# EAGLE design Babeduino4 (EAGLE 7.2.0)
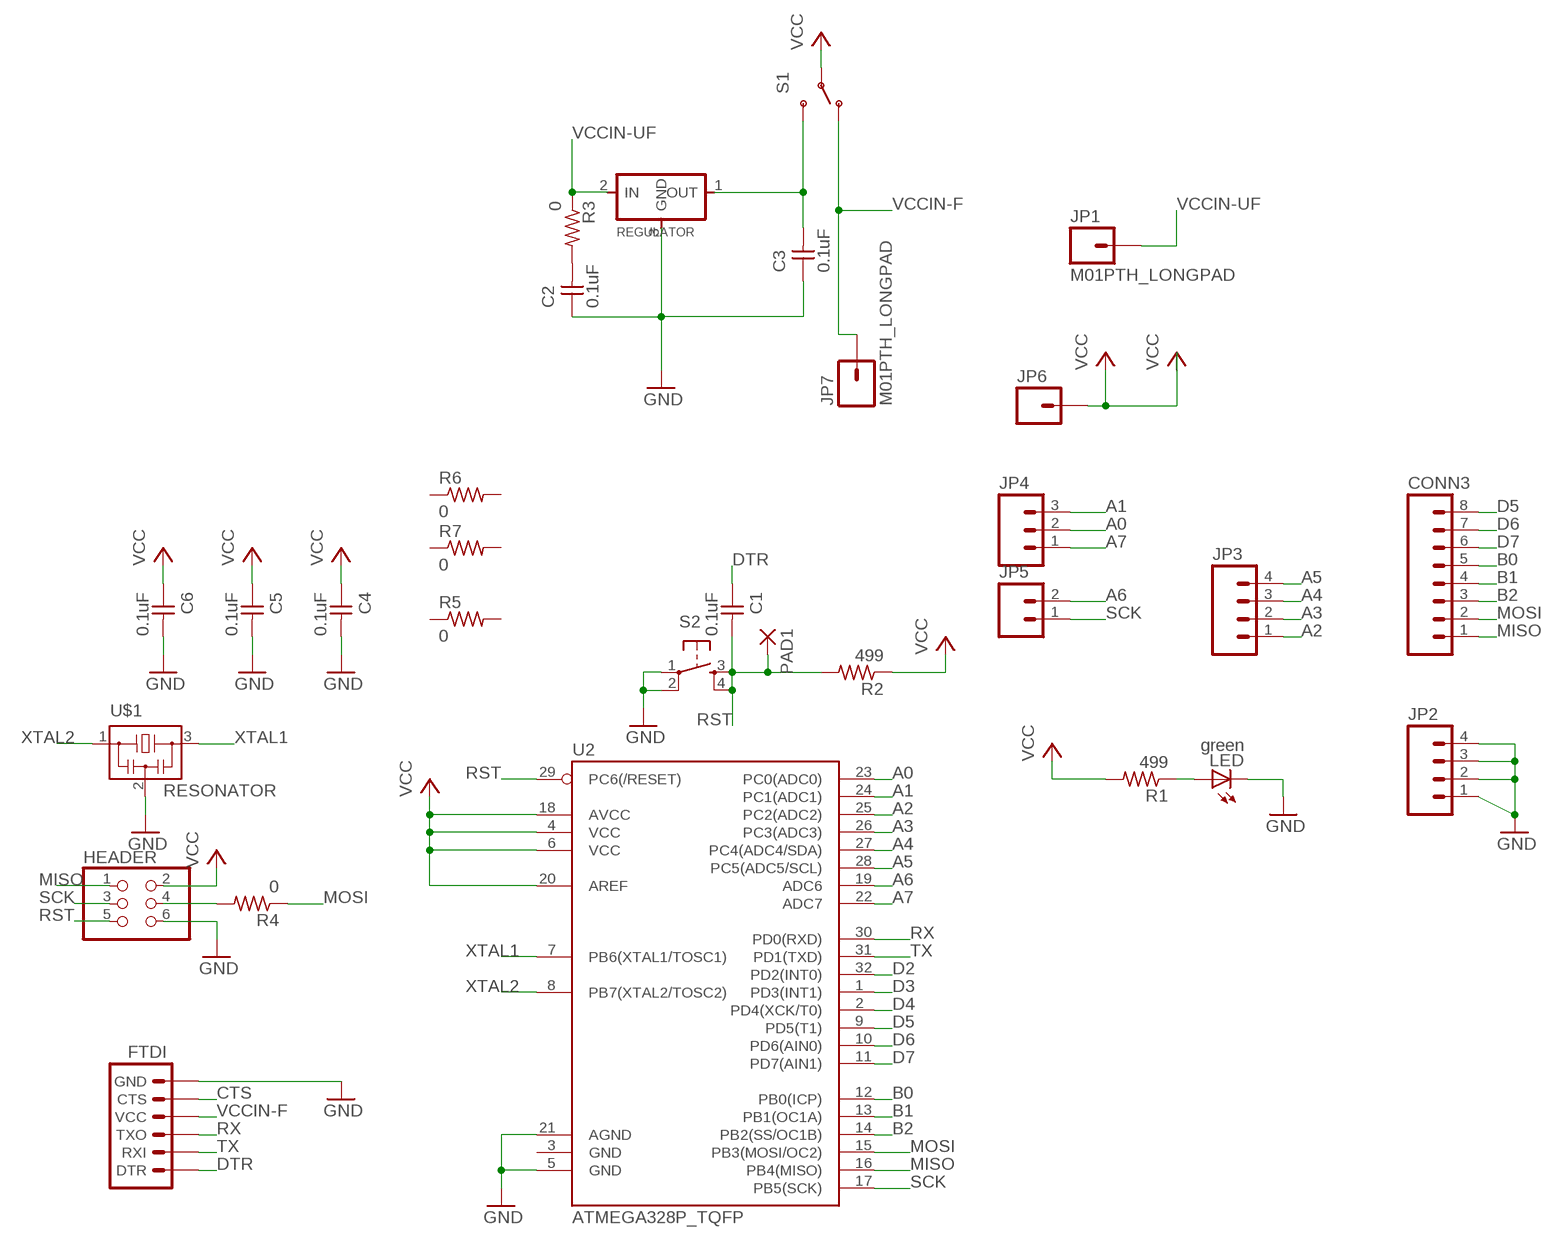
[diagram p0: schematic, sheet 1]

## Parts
C1  0.1uF  UNPOLARIZED_CAPACITOR1206  [1206]
C2  0.1uF  UNPOLARIZED_CAPACITOR1206  [1206]
C3  0.1uF  UNPOLARIZED_CAPACITOR1206  [1206]
C4  0.1uF  UNPOLARIZED_CAPACITOR1206  [1206]
C5  0.1uF  UNPOLARIZED_CAPACITOR1206  [1206]
C6  0.1uF  UNPOLARIZED_CAPACITOR1206  [1206]
CONN3  M08LONGPADS  [1X08_LONGPADS]
FTDI  ARDUINO_SERIAL_PROGRAMSMD  [1X06-SMD]
HEADER  PINHD-2X3-SMD  [2X03SMD]
JP1  M01PTH_LONGPAD  [1X01_LONGPAD]
JP2  M04LONGPADS  [1X04_LONGPADS]
JP3  M04LONGPADS  [1X04_LONGPADS]
JP4  M03LONGPADS  [1X03_LONGPADS]
JP5  M02  [1X02_LONGPADS]
JP6  M01PTH_LONGPAD  [1X01_LONGPAD]
JP7  M01PTH_LONGPAD  [1X01_LONGPAD]
LED  green  LED1206  [1206]
PAD1  WIREPAD2,54/0,9  [2,54/0,9]
R1  499  RESISTOR1206  [1206]
R2  499  RESISTOR1206  [1206]
R3  0  RESISTOR1206  [1206]
R4  0  RESISTOR1206  [1206]
R5  0  RESISTOR1206  [1206]
R6  0  RESISTOR1206  [1206]
R7  0  RESISTOR1206  [1206]
REGULATOR  REGULATORSOT23  [SOT23]
S1  SWITCH-SPDTSMD2  [SWITCH-SPDT-SMD]
S2  6MM_SWITCH6MM_SWITCH  [6MM_SWITCH]
U2  ATMEGA328P_TQFP  [TQFP32-08]
U$1  RESONATOR  [EFOBM]

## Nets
A0: JP4.2 U2.23(PC0(ADC0))
A1: JP4.3 U2.24(PC1(ADC1))
A2: JP3.1 U2.25(PC2(ADC2))
A3: JP3.2 U2.26(PC3(ADC3))
A4: JP3.3 U2.27(PC4(ADC4/SDA))
A5: JP3.4 U2.28(PC5(ADC5/SCL))
A6: JP5.2 U2.19(ADC6)
A7: JP4.1 U2.22(ADC7)
B0: CONN3.5 U2.12(PB0(ICP))
B1: CONN3.4 U2.13(PB1(OC1A))
B2: CONN3.3 U2.14(PB2(SS/OC1B))
CTS: FTDI.5(CTS)
D2: U2.32(PD2(INT0))
D3: U2.1(PD3(INT1))
D4: U2.2(PD4(XCK/T0))
D5: CONN3.8 U2.9(PD5(T1))
D6: CONN3.7 U2.10(PD6(AIN0))
D7: CONN3.6 U2.11(PD7(AIN1))
DTR: C1.1 FTDI.1(DTR)
GND: C2.1 C3.1 C4.2 C5.2 C6.2 FTDI.6(GND) HEADER.6 JP2.1 JP2.2 JP2.3 JP2.4 LED.2(C) REGULATOR.3(GND) S2.1(P) S2.2(P1) U2.5(GND) U2.21(AGND) U$1.2
MISO: CONN3.1 HEADER.1 U2.16(PB4(MISO))
MOSI: CONN3.2 R4.1 U2.15(PB3(MOSI/OC2))
N$1: LED.1(A) R1.1
N$2: HEADER.4 R4.2
N$3: C2.2 R3.2
N$4: C3.2 REGULATOR.1(OUT) S1.3(S)
RST: C1.2 HEADER.5 PAD1.1(P) R2.2 S2.3(S) S2.4(S1) U2.29(PC6(/RESET))
RX: FTDI.3(TXO) U2.30(PD0(RXD))
SCK: HEADER.3 JP5.1 U2.17(PB5(SCK))
TX: FTDI.2(RXI) U2.31(PD1(TXD))
VCC: C4.1 C5.1 C6.1 HEADER.2 JP6.1 R1.2 R2.1 S1.2(P) U2.4(VCC) U2.6(VCC) U2.18(AVCC) U2.20(AREF)
VCCIN-F: FTDI.4(VCC) JP7.1 S1.1(O)
VCCIN-UF: JP1.1 R3.1 REGULATOR.2(IN)
XTAL1: U2.7(PB6(XTAL1/TOSC1)) U$1.3
XTAL2: U2.8(PB7(XTAL2/TOSC2)) U$1.1
Unconnected: R5.1 R5.2 R6.1 R6.2 R7.1 R7.2 U2.3(GND)

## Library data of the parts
C1-C6 = 01_FAB_Hello:UNPOLARIZED_CAPACITOR: unpolarized_capacitor
CONN3 = 01_SparkFun:M08: Header 8 Standard 8-pin 0.1" header. Use with straight break away headers (SKU : PRT-00116), right angle break away headers (PRT-00553), swiss pins (PRT-00743), machine pins (PRT-00117), and female headers (PRT-00115).
FTDI = SparkFun-Connectors:ARDUINO_SERIAL_PROGRAM: FTDI connector footprints; PROD_ID: CONN-08971
HEADER = 01_FAB_Hello:PINHD-2X3-SMD: PIN HEADER
JP1 JP6 JP7 = 01_SparkFun:M01: Header 1
JP2 JP3 = 01_SparkFun:M04: Header 4 Standard 4-pin 0.1" header. Use with straight break away headers (SKU : PRT-00116), right angle break away headers (PRT-00553), swiss pins (PRT-00743), machine pins (PRT-00117), and female headers (PRT-00115). Molex polarized connector foot print use with SKU : PRT-08231 with associated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
JP4 = SparkFun-Connectors:M03: Header 3 Standard 3-pin 0.1" header. Use with straight break away headers (SKU : PRT-00116), right angle break away headers (PRT-00553), swiss pins (PRT-00743), machine pins (PRT-00117), and female headers (PRT-00115). Molex polarized connector foot print use with SKU : PRT-08232 with associated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
JP5 = 01_SparkFun:M02: Header 2
LED = 01_FAB_Hello:LED
PAD1 = wirepad:WIREPAD: Wire PAD connect wire on PCB
R1-R7 = 01_FAB_Hello:RESISTOR
REGULATOR = 01_fab:REGULATOR
S1 = SparkFun-Electromechanical:SWITCH-SPDT: SPDT Switch Simple slide switch, Spark Fun Electronics SKU : COM-00102 DPDT SMT slide switch, AYZ0202, SWCH-08179
S2 = 01_FAB_Hello:6MM_SWITCH: OMRON SWITCH
U2 = SparkFun-DigitalIC:ATMEGA328P_TQFP; PROD_ID: IC-09069
U$1 = 01_fab:RESONATOR

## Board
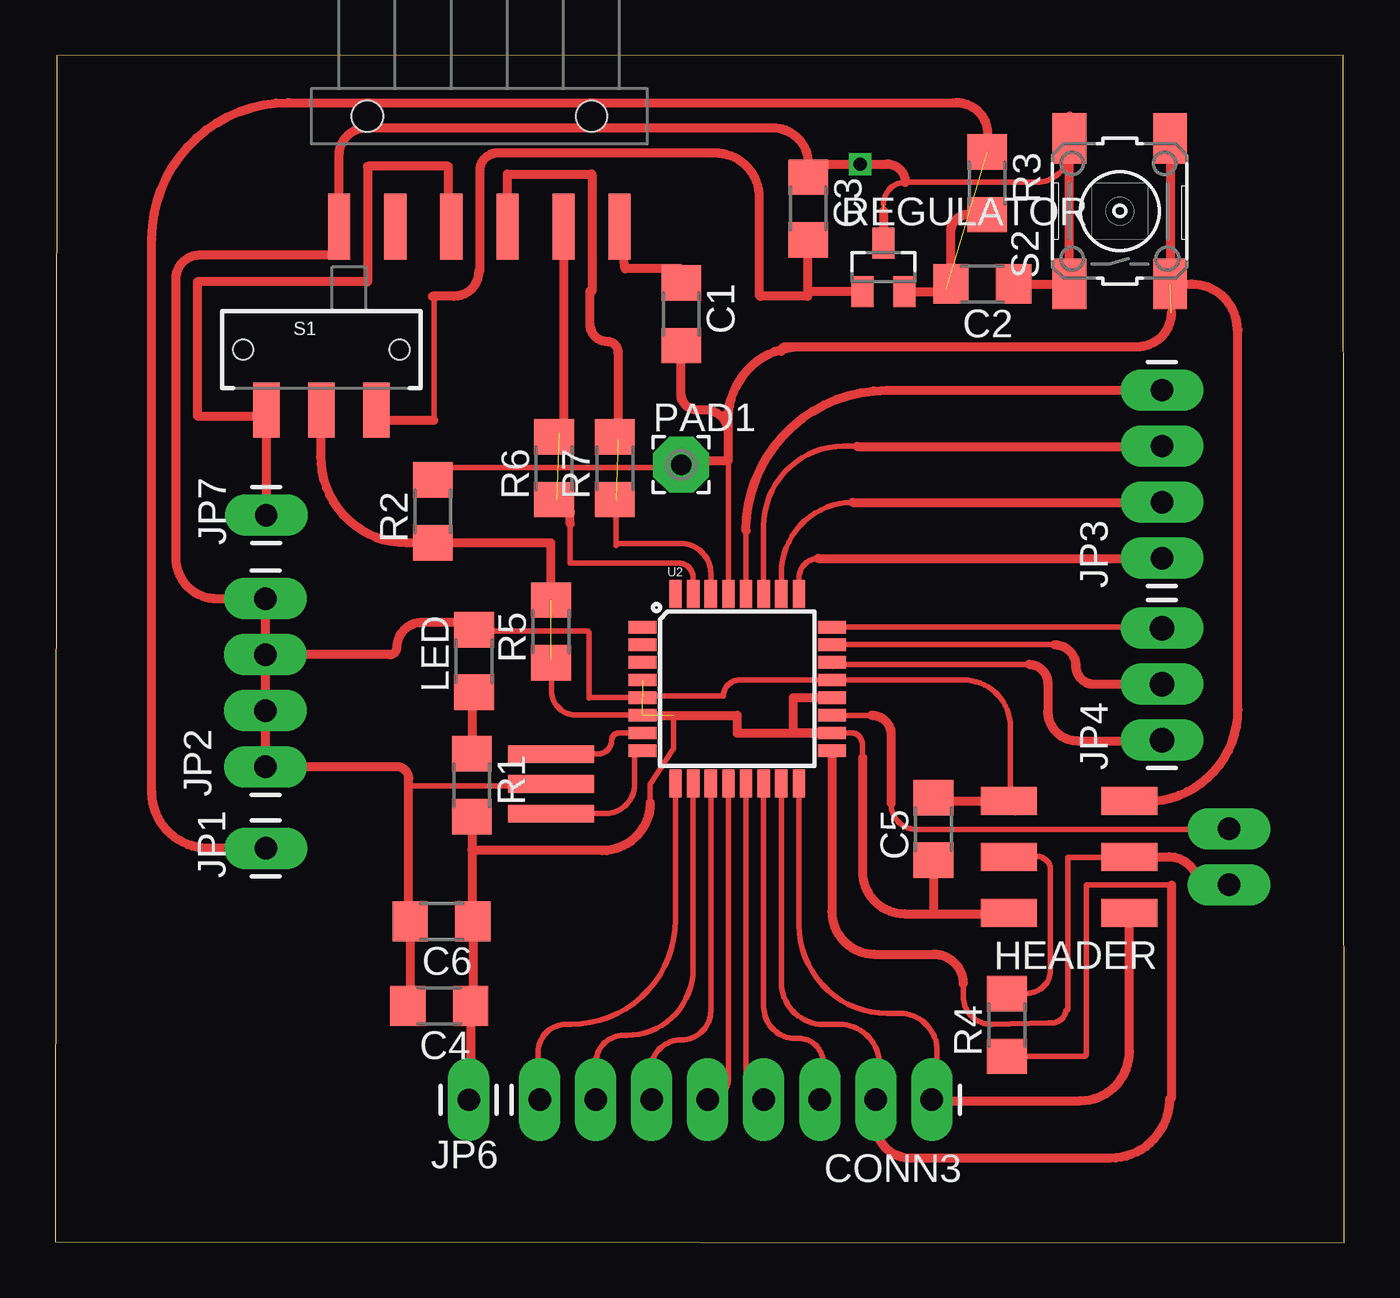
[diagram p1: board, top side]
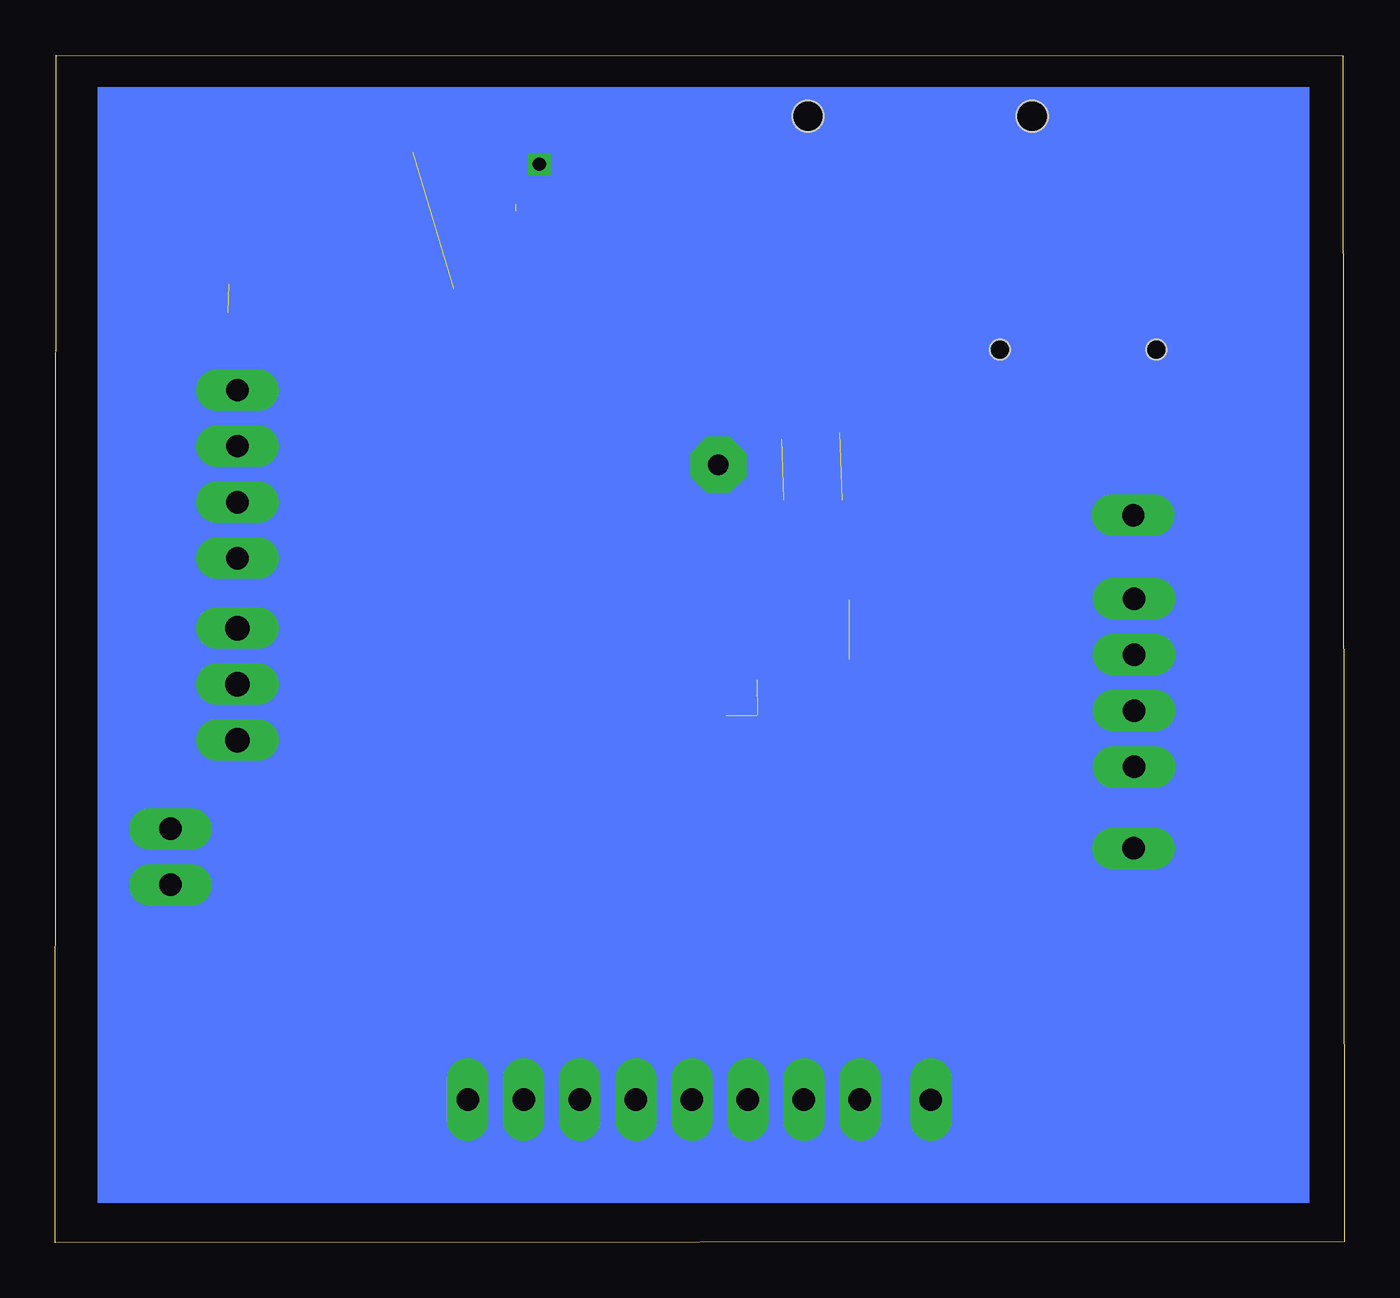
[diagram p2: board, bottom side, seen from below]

Size 58.45 x 53.84 mm. Coordinates in mm from the lower left corner, seen from the top.
Outline: 0,0.04 58.45,0 58.39,53.84 0.08,53.81 0,0.04
Copper layers (1*16): Top 0.035mm / dielectric 1.5mm / Bottom 0.035mm
Design rules "fabmodule": minimum track width 10mil, minimum drill 0.4mm, track to track 0.42mm, track to pad 0.42mm, pad to pad 0.42mm, via to via 0.42mm, smd to smd 0.42mm, copper to edge 40mil, drill to drill 0.8mm, minimum pad ring 10mil, minimum via ring 8mil, stop-mask expansion 4mil, vias tented up to drill 0mil, thermal gap 10mil

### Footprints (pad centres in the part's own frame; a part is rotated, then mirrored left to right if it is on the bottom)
1206 = smd 1.6 x 1.803: 1 -1.422,0; 2 1.422,0
1X08_LONGPADS = drill 1.016 pad 1.88 long: 1 0,0; 2 2.54,0; 3 5.08,0; 4 7.62,0; 5 10.16,0; 6 12.7,0; 7 15.24,0; 8 17.78,0
1X06-SMD = smd 1 x 3: 1 -6.35,5; 2 -3.81,5; 3 -1.27,5; 4 1.27,5; 5 3.81,5; 6 6.35,5 | hole 1.4: -5.08,0; 5.08,0
2X03SMD = smd 2.54 x 1.27: 1 -2.54,2.54; 2 2.92,2.54; 3 -2.54,0; 4 2.92,0; 5 -2.54,-2.54; 6 2.92,-2.54
1X01_LONGPAD = drill 1.016 pad 1.88 long: 1 0,0
1X04_LONGPADS = drill 1.016 pad 1.88 long: 1 0,0; 2 2.54,0; 3 5.08,0; 4 7.62,0
1X03_LONGPADS = drill 1.118 pad 1.88 long: 1 0,0; 2 2.54,0; 3 5.08,0
1X02_LONGPADS = drill 1.016 pad 1.88 long: 1 0,0; 2 2.54,0
2,54/0,9 = drill 0.914 pad 2.54 octagon: 1 0,0
SOT23 = smd 1 x 1.4: 1 -0.95,-1.1; 2 0.95,-1.1; 3 0,1.1
SWITCH-SPDT-SMD = smd 1.2 x 2.5: 1 -2.5,-2.75; 2 0,-2.75; 3 2.5,-2.75 | hole 0.9: -3.55,0; 3.55,0
6MM_SWITCH = smd 2.286 x 1.524: 1 -3.302,2.286; 2 3.302,2.286; 3 -3.302,-2.286; 4 3.302,-2.286
TQFP32-08 = smd 1.27 x 0.559: 1 -4.293,2.8; 2 -4.293,2; 3 -4.293,1.2; 4 -4.293,0.4; 5 -4.293,-0.4; 6 -4.293,-1.2; 7 -4.293,-2; 8 -4.293,-2.8; 17 4.293,-2.8; 18 4.293,-2; 19 4.293,-1.2; 20 4.293,-0.4; 21 4.293,0.4; 22 4.293,1.2; 23 4.293,2; 24 4.293,2.8 | smd 0.559 x 1.27: 9 -2.8,-4.293; 10 -2,-4.293; 11 -1.2,-4.293; 12 -0.4,-4.293; 13 0.4,-4.293; 14 1.2,-4.293; 15 2,-4.293; 16 2.8,-4.293; 25 2.8,4.293; 26 2,4.293; 27 1.2,4.293; 28 0.4,4.293; 29 -0.4,4.293; 30 -1.2,4.293; 31 -2,4.293; 32 -2.8,4.293
EFOBM = smd 0.8 x 3.9: 1 -1.35,0; 2 0,0; 3 1.35,0

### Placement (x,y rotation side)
C1  28.39,42.09 270 top
C2  42.03,43.46 180 top
C3  34.15,46.89 270 top
C4  17.41,10.74 180 top
C5  39.82,18.76 90 top
C6  17.52,14.56 180 top
CONN3  39.75,6.48 180 top
FTDI  19.23,51.07 180 top
HEADER  46.17,17.49 180 top
JP1  9.55,17.88 90 top
JP2  9.54,21.58 90 top
JP3  50.18,31.04 90 top
JP4  50.18,22.78 90 top
JP5  53.22,16.22 90 top
JP6  18.76,6.47 180 top
JP7  9.57,32.98 90 top
LED  18.99,26.37 90 top
PAD1  28.39,35.27 0 top
R1  18.89,20.74 270 top
R2  17.12,33.16 90 top
R3  42.26,48.03 270 top
R4  43.15,9.87 90 top
R5  22.48,27.71 90 top
R6  22.62,35.11 90 top
R7  25.38,35.11 90 top
REGULATOR  37.55,44.22 0 top
S1  12.07,40.49 0 top
S2  48.27,46.77 90 top
U2  30.93,25.11 0 top
U$1  22.49,20.8 90 top

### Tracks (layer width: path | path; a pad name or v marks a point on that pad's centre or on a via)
A0
  Top 0.254: U2.23 45.31,27.11
  Top 0.406: 45.31,27.11 arc-90 46.28,26.14 arc90 47.1,25.32 JP4.2
A1
  Top 0.254: U2.24 50.13,27.91 arc-90 JP4.3
  Top 0.406: 50.13,27.91 arc-90 JP4.3
A2
  Top 0.254: U2.25 33.73,30.14 arc-90 34.6,31.02
  Top 0.406: 34.6,31.02 50.42,31.02 arc-90 50.64,30.8 50.41,30.8 arc-90 JP3.1
A3
  Top 0.254: U2.26 32.93,30.33 arc-90 36.15,33.56
  Top 0.406: 36.15,33.56 50.17,33.56 arc90 JP3.2
A4
  Top 0.254: U2.27 32.13,32.49 arc-90 35.75,36.11 36.36,36.11 arc-90 36.37,36.1
  Top 0.406: 36.37,36.1 50.17,36.1 arc90 JP3.3
A5
  Top 0.254: U2.28 31.33,32.26
  Top 0.406: 31.33,32.26 arc-90 37.71,38.65 50.17,38.65 arc90 JP3.4
A6
  Top 0.254: 37.9,19.93 37.9,19.89 arc90 39.07,18.73 53.18,18.73 arc90 JP5.2 | U2.19 37.03,23.91
  Top 0.406: JP5.2 arc90 JP5.2 arc-90 53.18,18.73 | 37.03,23.91 arc-90 37.9,23.04 37.9,19.93
A7
  Top 0.254: 35.31,26.21 44.16,26.21
  Top 0.406: U2.22 arc90 35.31,26.21 | 44.16,26.21 arc-90 45,25.37 45,24.1 arc90 46.35,22.75 50.15,22.75 arc90 JP4.1
B0
  Top 0.254: U2.12 30.53,7.42 arc-90 CONN3.5
B1
  Top 0.254: U2.13 31.33,7.28 arc90 CONN3.4
B2
  Top 0.254: U2.14 32.13,10.69 arc90 33.56,9.26 33.7,9.26 arc-90 34.83,8.13 34.83,6.65 arc-90 CONN3.3
  Top 0.406: 34.9,6.72 arc-90 CONN3.3
D5
  Top 0.254: U2.9 28.13,14.64 arc-90 23.38,9.9 23.17,9.9 arc90 21.9,8.63 21.9,6.55 arc90 CONN3.8
D6
  Top 0.254: U2.10 28.93,12.4 arc-90 25.93,9.4 25.78,9.4 arc90 24.51,8.13 CONN3.7 arc-90 CONN3.7
D7
  Top 0.254: U2.11 29.73,10.52 arc-90 28.4,9.19 | 28.4,9.19 | 28.4,9.19 arc90 26.99,7.78 26.99,6.54 arc90 CONN3.6
DTR
  Top 0.406: C1.1 28.39,44.16 25.85,44.16 FTDI.1
GND  (via drill 0.6)  (1 unrouted)
  Top 0.254: HEADER.6 arc90 43.31,20.09 43.31,23.39 arc90 41.19,25.51 U2.21 31.03,25.51 arc90 30.3,24.77 26.7,24.77 arc90 U2.5 | 37.56,47.08 arc-90 38.55,48.07 44.48,48.07 arc90 45.99,49.58 | U2.5 arc-90 26.61,24.69 | LED.2 arc-90 LED.2 arc90 19.05,27.73 24.09,27.73 arc-90 24.2,27.63 24.2,24.69 arc-90 24.22,24.71 U2.5 | U2.5 arc-90 26.67,24.74 | U$1.2 arc-90 22.4,20.71 16.03,20.71
  Top 0.406: C5.2 39.82,20.03 HEADER.6 arc-90 43.56,19.71 43.56,19.57 arc-90 43.28,19.86 | S2.1 arc90 S2.1 | S2.1 45.99,49.58 S2.2 arc90 S2.2 45.99,51.08 | 37.56,46.77 REGULATOR.3 arc-90 REGULATOR.3 37.54,45.32 | C2.1 S2.1 | C4.2 arc90 16.1,10.85 C6.2 arc-90 16.03,14.63 16.03,20.71 16.03,21.04 arc90 15.49,21.58 JP2.1 JP2.2 JP2.3 | LED.2 18.99,28.1 arc90 18.97,28.12 16.63,28.12 arc90 15.49,26.97 arc-90 15.17,26.66 JP2.3 | JP2.3 JP2.4 7.33,29.2 arc-90 5.47,31.06 5.47,43.69 arc-90 6.56,44.78 12.99,44.78 arc90 13.06,44.85 arc90 13.15,44.94 13.15,46.23 arc-90 12.99,46.07 FTDI.6 arc-90 12.87,46.08 12.87,49.29 arc-90 14.13,50.55 32.53,50.55 arc-90 34.15,48.93 | U2.21 arc-90 35.16,25.45 | 34.06,48.63 arc90 34.26,48.43 arc-90 C3.1 34.15,48.93 | 34.15,48.93 arc90 34.18,48.9 v36.5,48.9 37.72,48.9 arc-90 38.55,48.07
MISO
  Top 0.254: U2.16 33.73,14.39 arc90 37.73,10.39 38.29,10.39 arc-90 39.99,8.7 39.99,6.73 arc-90 CONN3.1
  Top 0.406: CONN3.1 arc90 39.92,6.66 arc90 40.14,6.44 46.49,6.44 arc90 48.71,8.65 HEADER.1
MOSI
  Top 0.254: R4.1 46.64,8.45 arc90 46.75,8.55 46.75,16.16 arc-90 46.8,16.22 50.61,16.22 | U2.15 32.93,11.8 arc90 34.83,9.9 35.54,9.9 arc-90 37.38,8.06 37.38,6.65 arc-90 CONN3.2
  Top 0.406: 37.3,6.58 arc-90 CONN3.2 37.21,5.41 arc90 38.79,3.82 47.84,3.82 arc90 50.52,6.51 arc90 50.61,6.6 50.61,16.22
N$1
  Top 0.406: LED.1 arc90 18.89,24.85 R1.1
N$2
  Top 0.254: HEADER.4 44.25,17.49 arc-90 45.13,17.03 45.13,12.44 arc-90 44.14,11.31 43.17,11.31 arc90 R4.2
N$3
  Top 0.406: C2.2 40.61,45.81 arc-90 41.42,46.63 42.19,46.63 arc-90 R3.2
N$4
  Top 0.254: 17.17,37.28 17.17,42.8 arc-90 17.28,42.91
  Top 0.406: C3.2 34.12,45.47 34.12,43.12 | 34.12,43.12 34.12,42.91 31.99,42.91 | REGULATOR.1 34.12,43.12 | 31.99,42.91 31.96,42.91 | 17.17,37.28 14.57,37.28 | 14.3,37.28 14.57,37.28 | 14.57,37.28 S1.3 | 17.11,42.91 17.28,42.91 18.09,42.91 arc90 19.2,44.03 arc-90 19.25,44.07 19.25,48.59 arc-90 20.06,49.4 29.92,49.4 arc-90 31.93,47.39 31.93,42.96 arc90 31.99,42.91
RST  (1 unrouted)
  Top 0.254: U2.29 30.53,35.39 arc90 30.45,35.47 | PAD1.1 arc-90 28.07,35.14 16.86,35.14 arc-90 17.12,35.08 R2.2
  Top 0.406: S2.4 S2.3 51.52,43.47 arc-90 53.58,41.4 arc-90 53.63,41.35 53.63,24.17 arc-90 49.46,20 48.74,20 arc-90 HEADER.5 | 30.53,36.7 30.53,35.47 30.45,35.47 28.59,35.47 arc90 PAD1.1 | 30.53,36.7 arc90 29.47,37.75 29.12,37.75 arc-90 28.38,38.49 C1.2 arc-90 C1.2 | 30.53,36.7 30.53,37.34 | 30.53,37.34 arc-90 33.81,40.62 | 33.81,40.62 49.06,40.62 arc90 50.62,42.18 | 32.92,40.41 arc-90 33.13,40.62 33.81,40.62 | 30.53,37.34 arc-90 30.41,37.46 arc-90 30.35,37.51
RX  (1 unrouted)
  Top 0.254: U2.30 29.73,30.34 arc90 28.37,31.69 25.52,31.69 arc90 25.42,31.6 25.42,33.67
  Top 0.406: FTDI.3 20.5,48.45 | 20.5,48.45 | 20.5,48.45 24.34,48.45 24.34,43.13 24.24,43.13 24.24,41.65 arc90 25.03,40.86 arc-90 25.52,40.37 25.52,36.43
SCK
  Top 0.254: 41.17,11.73 41.17,11.17 arc90 42.45,9.9 45.06,9.97 arc90 45.84,10.53 arc90 45.93,10.62 45.93,17.47 arc90 45.95,17.46 48.67,17.46 arc90 HEADER.3
  Top 0.406: HEADER.3 50.51,17.49 arc-90 51.82,16.18 53.18,16.18 arc90 JP5.1 | U2.17 35.22,15 arc90 37.15,13.08 39.83,13.08 arc-90 41.17,11.73
TX  (1 unrouted)
  Top 0.254: U2.31 28.93,30.16 arc90 28.28,30.81 23.35,30.81 23.35,32.58
  Top 0.406: FTDI.2 23.04,36.9 arc-90 22.86,36.72 | 23.35,32.58 23.35,33.08 arc90 22.76,33.67
VCC  (3 unrouted)
  Top 0.254: 28.05,23.91 28.05,22.4 26.98,20.77 26.98,19.95 | 35.47,23.11 36.1,23.11 arc-90 36.6,22.61 36.6,21.98 arc90 36.6,21.98 | 26.62,23.92 arc-90 U2.6 arc90 26.62,23.92 | 26.62,23.92 23.6,23.92 arc-90 22.51,25.01 22.51,26.37 arc90 22.46,26.43
  Top 0.406: U2.6 30.93,23.91 30.93,23.11 U2.18 | U2.18 33.47,23.11 33.47,24.71 U2.20 | U2.18 35.47,23.11 | 36.6,21.98 36.6,16.82 arc90 38.51,14.91 39.86,14.91 | 39.86,14.91 43.21,14.91 arc90 HEADER.2 | C5.1 39.82,14.95 arc90 39.86,14.91 | R1.2 18.89,17.83 | 18.89,17.83 18.89,14.61 arc90 C6.1 18.94,10.85 arc-90 C4.1 18.83,6.93 arc-90 JP6.1 | 26.98,19.95 arc-90 24.8,17.77 18.95,17.77 arc-90 18.89,17.83 | 22.47,29.13 22.47,31.74 R2.1 15.94,31.74 arc-90 12.04,35.64 12.04,37.74 S1.2
VCCIN-F
  Top 0.406: FTDI.4 17.83,46.07 17.83,48.8 14.16,48.8 14.16,43.56 6.44,43.56 6.44,37.48 9.57,37.48 S1.1 JP7.1 arc90 JP7.1
VCCIN-UF  (1 unrouted)
  Top 0.406: 42.04,49.63 arc90 R3.1 arc90 42.28,49.47 42.28,50.28 arc90 40.86,51.69 10.57,51.69 arc90 4.39,45.51 4.39,20.42 arc90 6.93,17.88 JP1.1 | REGULATOR.2 40.48,43.12 arc90 40.49,43.13 | 40.49,43.13 | 40.49,43.13 arc90 40.39,43.24
XTAL1
  Top 0.254: U2.7 25.56,23.11 arc90 25.24,22.78 arc-90 24.6,22.15 U$1.3
XTAL2
  Top 0.254: U$1.1 arc-90 22.5,19.46 24.96,19.46 arc90 26.27,20.77 26.27,21.94 arc-90 U2.8
(copper drawn outside any net)
  shapes: Bottom area x1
